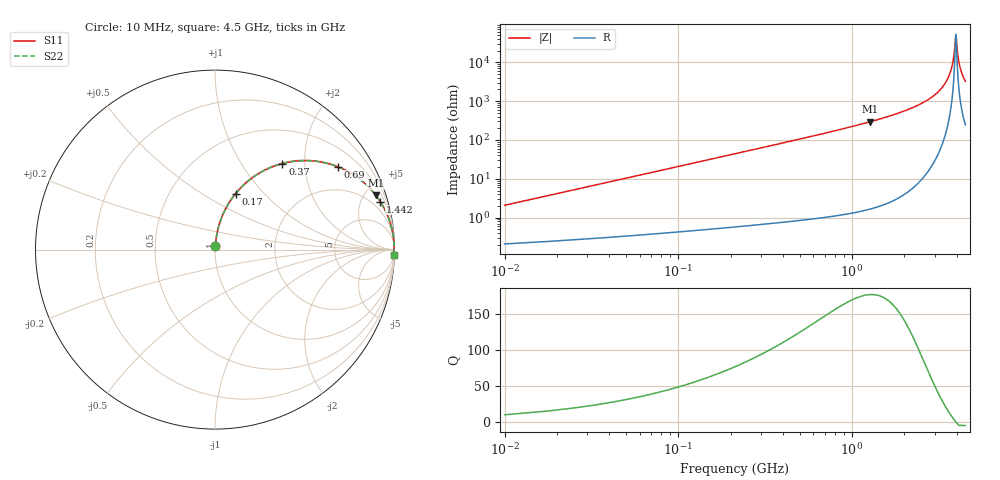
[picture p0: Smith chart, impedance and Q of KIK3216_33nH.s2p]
!version-2
!date-01.2022
!Series
# MHz S RI R 50
!Freq ReS11 ImS11 ReS21 ImS21 ReS12 ImS12 ReS22 ImS22
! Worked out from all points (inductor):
!   563 points, 10 MHz to 4.5 GHz, reference 50 ohm
!   read as one part in series: L = 33 nH near 26 MHz
!   highest Q = 177 at 1.274 GHz (marker M1), where L = 36.8 nH
!   self-resonance near 3.962 GHz
!   S11 on the Smith chart (normalised r, x): 10 MHz: 1.00, +0.04; 170 MHz: 1.01, +0.71; 370 MHz: 1.01, +1.55; 690 MHz: 1.02, +2.95; 1.442 GHz: 1.04, +6.89; 4.5 GHz: 6, -65
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10  0.00253 0.0206  0.9975 -0.0206  0.9975 -0.0206  0.00253 0.0206
42  0.0106 0.0859  0.9894 -0.0859  0.9894 -0.0859  0.0106 0.0859
66  0.0219 0.1334  0.9781 -0.1334  0.9781 -0.1334  0.0219 0.1334
106  0.0499 0.2081  0.9501 -0.2081  0.9501 -0.2081  0.0499 0.2081
170  0.1145 0.3111  0.8855 -0.3111  0.8855 -0.3111  0.1145 0.3111
370  0.3757 0.4796  0.6243 -0.4796  0.6243 -0.4796  0.3757 0.4796
690  0.684 0.4615  0.316 -0.4615  0.316 -0.4615  0.684 0.4615
762  0.7278 0.4419  0.2722 -0.4419  0.2722 -0.4419  0.7278 0.4419
1274  0.8953 0.3034  0.1047 -0.3034  0.1047 -0.3034  0.8953 0.3034
1442  0.921 0.2669  0.079 -0.2669  0.079 -0.2669  0.921 0.2669
1514  0.9298 0.2526  0.0702 -0.2526  0.0702 -0.2526  0.9298 0.2526
2258  0.9784 0.1411  0.0216 -0.1411  0.0216 -0.1411  0.9784 0.1411
3010  0.994 0.0675  0.00597 -0.0675  0.00597 -0.0675  0.994 0.0675
3474  0.9974 0.0323  0.00265 -0.0323  0.00265 -0.0323  0.9974 0.0323
3754  0.998 0.0134  0.00195 -0.0134  0.00195 -0.0134  0.998 0.0134
3858  0.9981 0.00679  0.00189 -0.00679  0.00189 -0.00679  0.9981 0.00679
3946  0.9981 0.00133  0.0019 -0.00133  0.0019 -0.00133  0.9981 0.00133
3970  0.9981 -0.000139  0.00192 0.000139  0.00192 0.000139  0.9981 -0.000139
4066  0.998 -0.00592  0.00202 0.00592  0.00202 0.00592  0.998 -0.00592
4154  0.9978 -0.0111  0.00218 0.0111  0.00218 0.0111  0.9978 -0.0111
4298  0.9975 -0.0194  0.00254 0.0194  0.00254 0.0194  0.9975 -0.0194
4500  0.9967 -0.0305  0.00326 0.0305  0.00326 0.0305  0.9967 -0.0305
